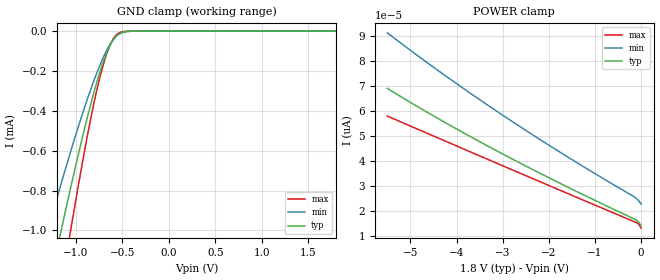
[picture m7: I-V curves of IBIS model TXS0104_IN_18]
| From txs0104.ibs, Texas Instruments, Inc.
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[Model]   TXS0104_IN_18
Model_type  Input
Vinl=0.5775
Vinh=1.2675
| variable   typ   min   max
C_comp   0.22pF   0.17pF   0.26pF
[Temperature Range]   40   100   -40
| Ambient temperature   25   85   -40
[Voltage range]   1.8   1.65   1.95
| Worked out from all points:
|   GND clamp passes 1 mA (typ) near -1.16 V on its own axis
[GND Clamp]
| TXS0104_IN_18
|   Voltage   I(typ)   I(min)   I(max)
-5.5V     -12.44mA   -9.732mA   -15.69mA
-1.3V     -1.314mA   -1.001mA   -1.704mA
-1.165V   -1.017mA   -777.6uA   -1.309mA
-1.085V   -847.2uA   -650.4uA   -1.082mA
-1.045V   -764.4uA   -588.4uA   -970.6uA
-875mV    -431.7uA   -340.5uA   -524uA
-800mV    -299.2uA   -242.1uA   -350.2uA
-740mV    -203.5uA   -170.5uA   -230.9uA
-635mV    -74.55uA   -68.66uA   -73.26uA
-550mV    -20.17uA   -19.87uA   -13.42uA
-400mV    -564.5nA   -736.8nA   -109.2nA
1.8V      14.22pA    25.69pA    10.81pA
[POWER Clamp]
| TXS0104_IN_18
|   Voltage   I(typ)   I(min)   I(max)
-5.5V     69pA       91.19pA    57.95pA
-4.395V   56.91pA    76.09pA    49.16pA
-3.24V    45.16pA    61.27pA    40.01pA
-1.77V    31.22pA    43.68pA    28.43pA
-130mV    16.66pA    25.44pA    15.62pA
-55mV     15.63pA    24.2pA     14.78pA
-95.1fV   14.22pA    22.83pA    13.18pA
